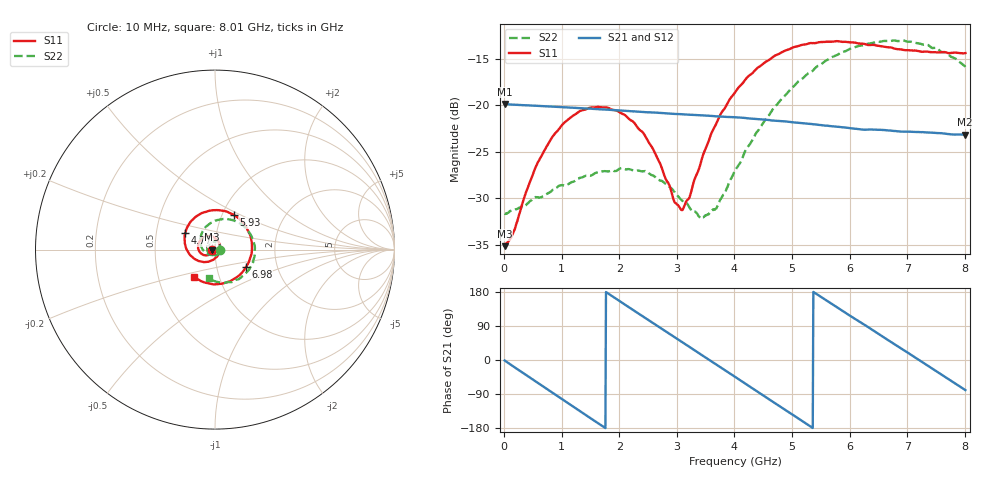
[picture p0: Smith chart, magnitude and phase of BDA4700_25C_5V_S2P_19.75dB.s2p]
!Agilent Technologies,E5071B,MY42404982,A.09.10
!Date: Mon Oct 20 13:36:15 2025
!Data & Calibration Information:
!Freq	S11:SOLT2(ON)	S21:SOLT2(ON)	S12:SOLT2(ON)	S22:SOLT2(ON)
# Hz S RI R 50
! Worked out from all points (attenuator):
!   801 points, 10 MHz to 8.01 GHz, reference 50 ohm
!   highest |S21| = -19.84 dB at 10 MHz (marker M1); lowest = -23.1 dB at 8 GHz (marker M2)
!   lowest |S11| = -35.1 dB at 10 MHz (marker M3), VSWR 1.04, Z = 48.3 - j0.0988 ohm
!   |S11| at or under -10 dB: start of sweep to end of sweep
!   |S22| runs from -32.2 to -13.0 dB; largest |S21 - S12| = 0.00083
!   S11 on the Smith chart (normalised r, x): 10 MHz: 0.97, -0.00; 4.77 GHz: 0.71, +0.13; 5.93 GHz: 1.13, +0.46; 6.98 GHz: 1.38, -0.28; 8.01 GHz: 0.76, -0.24
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1e7  -0.0175 -0.00102  0.1018 -0.0022  0.1018 -0.00229  0.0262 -0.000892
1.6e8  -0.0184 -0.00953  0.0967 -0.0292  0.0967 -0.0293  0.0263 -0.00759
5.2e8  -0.034 -0.0284  0.0589 -0.0805  0.0589 -0.0806  0.0164 -0.0273
7.7e8  -0.0537 -0.0318  0.0183 -0.0971  0.0183 -0.0972  0.000679 -0.0339
1.35e9  -0.0941 0.00499  -0.0721 -0.0644  -0.0722 -0.0645  -0.0372 -0.0172
2.09e9  -0.0507 0.0733  -0.0787 0.0509  -0.0787 0.0509  -0.028 0.0359
2.42e9  -0.00891 0.0704  -0.0375 0.0843  -0.0376 0.0844  -0.00249 0.0442
2.68e9  0.0172 0.0478  0.00303 0.0913  0.00298 0.0913  0.0155 0.0367
2.96e9  0.0283 0.0107  0.0447 0.0782  0.0448 0.0781  0.0274 0.0205
3.1e9  0.0258 -0.00941  0.0621 0.0647  0.0619 0.0649  0.0294 0.00881
3.22e9  0.0194 -0.0254  0.0736 0.0503  0.0738 0.0503  0.0282 -3.93e-05
3.46e9  -0.00612 -0.0544  0.087 0.016  0.087 0.0159  0.0169 -0.0185
3.69e9  -0.0431 -0.0679  0.0854 -0.0188  0.0854 -0.0191  -0.00128 -0.028
4.01e9  -0.1024 -0.0579  0.0618 -0.0604  0.0618 -0.0603  -0.0351 -0.0271
4.77e9  -0.1657 0.091  -0.0419 -0.0711  -0.0416 -0.0713  -0.0811 0.0651
5.35e9  -0.0663 0.2062  -0.0794 -0.00231  -0.0794 -0.00253  -0.0139 0.1522
5.93e9  0.1033 0.1942  -0.0429 0.0628  -0.043 0.0627  0.1197 0.1549
6.68e9  0.2052 -0.00868  0.0458 0.0572  0.046 0.0572  0.2216 -0.00609
6.98e9  0.1718 -0.099  0.067 0.0274  0.0671 0.0271  0.2036 -0.0867
7.5e9  0.0338 -0.1902  0.0622 -0.0347  0.0621 -0.0348  0.0956 -0.1804
8e9  -0.1164 -0.1517  0.014 -0.0682  0.014 -0.0684  -0.034 -0.1591
8.01e9  -0.1191 -0.1499  0.0128 -0.0685  0.0128 -0.0686  -0.0362 -0.1572
